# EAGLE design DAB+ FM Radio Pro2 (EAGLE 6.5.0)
AUTHOR: JP Liew; PRODUCT_NAME: DAB+ FM Development Board Pro2; VERSION: 1.5
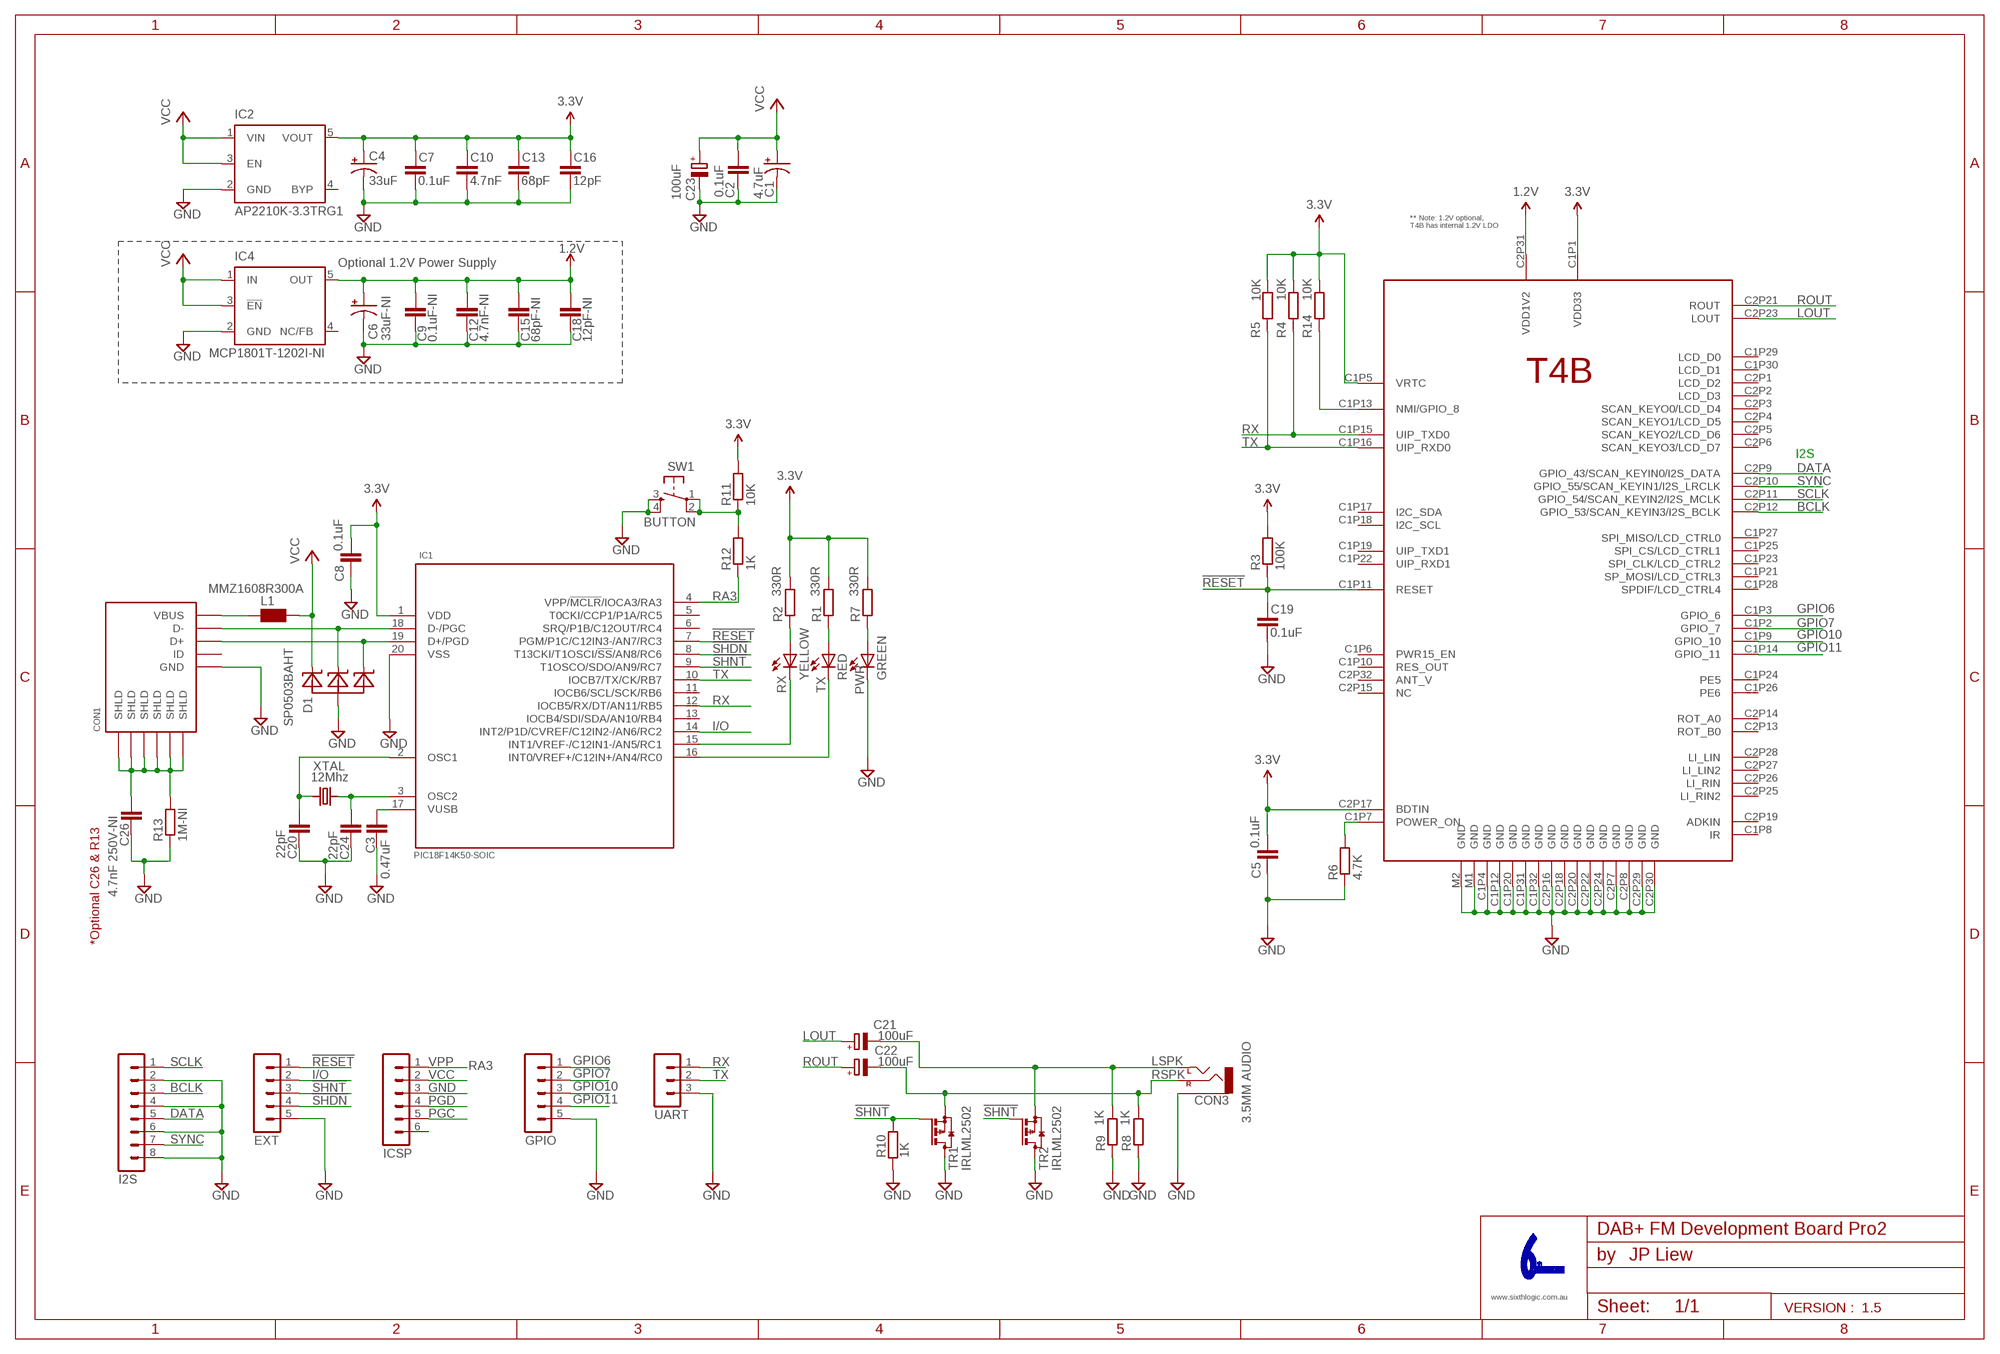
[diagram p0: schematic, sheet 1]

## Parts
C1  4.7uF  CAP_POL1206  [EIA3216]
C2  0.1uF  C-EUC0603  [C0603]
C3  0.47uF  C-EUC0603  [C0603]
C4  33uF  CAP_POL1206  [EIA3216]
C5  0.1uF  C-EUC0603  [C0603]
C6  33uF-NI  CAP_POL1206  [EIA3216]
C7  0.1uF  C-EUC0603  [C0603]
C8  0.1uF  C-EUC0603  [C0603]
C9  0.1uF-NI  C-EUC0603  [C0603]
C10  4.7nF  C-EUC0603  [C0603]
C12  4.7nF-NI  C-EUC0603  [C0603]
C13  68pF  C-EUC0603  [C0603]
C15  68pF-NI  C-EUC0603  [C0603]
C16  12pF  C-EUC0603  [C0603]
C18  12pF-NI  C-EUC0603  [C0603]
C19  0.1uF  C-EUC0603  [C0603]
C20  22pF  C-EUC0603  [C0603]
C21  100uF  CPOL-EUD  [PANASONIC_D]
C22  100uF  CPOL-EUD  [PANASONIC_D]
C23  100uF  CPOL-EUD  [PANASONIC_D]
C24  22pF  C-EUC0603  [C0603]
C26  4.7nF 250V-NI  C-EUC0603  [C0603]
CON1  MicroUSB  CONN_USB-4UCON-11071  [4UCON-11071]
CON3  3.5MM AUDIO  SJ-3523-SMT  [SJ-3523-SMT]
D1  SP0503BAHT  [SOT143]
EXT  MA05-1  [MA05-1]
GPIO  MA05-1  [MA05-1]
I2S  MA08-1  [MA08-1]
IC1  PIC18F14K50-SOIC  [SO20W]
IC2  AP2210K-3.3TRG1  [SOT23-5]
IC4  MCP1801T-1202I-NI  TPS77001  [SOT23-DBV]
ICSP  MA06-1  [MA06-1]
L1  MMZ1608R300A  WE-CBF_0603  [0603]
PWR  GREEN  LEDCHIP-LED0603  [CHIP-LED0603]
R1  330R  R-EU_R0603  [R0603]
R2  330R  R-EU_R0603  [R0603]
R3  100K  R-EU_R0603  [R0603]
R4  10K  R-EU_R0603  [R0603]
R5  10K  R-EU_R0603  [R0603]
R6  4.7K  R-EU_R0603  [R0603]
R7  330R  R-EU_R0603  [R0603]
R8  1K  R-EU_R0603  [R0603]
R9  1K  R-EU_R0603  [R0603]
R10  1K  R-EU_R0603  [R0603]
R11  10K  R-EU_R0603  [R0603]
R12  1K  R-EU_R0603  [R0603]
R13  1M-NI  R-EU_R0603  [R0603]
R14  10K  R-EU_R0603  [R0603]
RX  YELLOW  LEDCHIP-LED0603  [CHIP-LED0603]
SW1  BUTTON  SCHURTER_PUSH_BUTTON  [PUSH_BUTTON_SMD]
TR1  IRLML2502  DMP2305U  [SOT23]
TR2  IRLML2502  DMP2305U  [SOT23]
TX  RED  LEDCHIP-LED0603  [CHIP-LED0603]
U$1  T4B  T4B-SMD  [T4B-SMD]
UART  MA03-1  [MA03-1]
XTAL  12Mhz  CRYSTAL-HC49US  [HC49US-SMD]

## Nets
1.2V: C6.A(+) C9.1 C12.1 C15.1 C18.1 IC4.5(OUT) U$1.C2P31(VDD1V2)
3.3V: C4.A(+) C5.1 C7.1 C8.1 C10.1 C13.1 C16.1 IC1.1(VDD) IC2.5(VOUT) R1.2 R2.2 R3.2 R4.2 R5.2 R7.2 R11.2 R14.2 U$1.C1P1(VDD33) U$1.C1P5(VRTC) U$1.C2P17(BDTIN)
!RESET!: C19.1 EXT.1 IC1.7(PGM/P1C/C12IN3-/AN7/RC3) R3.1 U$1.C1P11(RESET)
!SHDN!: EXT.4 IC1.8(T13CKI/T1OSCI/!SS!/AN8/RC6)
!SHNT!: EXT.3 IC1.9(T1OSCO/SDO/AN9/RC7) R10.2 TR1.1(G) TR2.1(G)
BCLK: I2S.3 U$1.C2P12(GPIO_53/SCAN_KEYIN3/I2S_BCLK)
DATA: I2S.5 U$1.C2P9(GPIO_43/SCAN_KEYIN0/I2S_DATA)
GND: C1.C(-) C2.2 C3.2 C4.C(-) C5.2 C6.C(-) C7.2 C8.2 C9.2 C10.2 C12.2 C13.2 C15.2 C16.2 C18.2 C19.2 C20.2 C23.- C24.2 C26.2 CON1.GND CON3.1(SLEEVE) D1.1 EXT.5 GPIO.5 I2S.2 I2S.4 I2S.6 I2S.8 IC1.20(VSS) IC2.2(GND) IC4.2(GND) ICSP.3 PWR.C R6.1 R8.1 R9.1 R10.1 R13.1 SW1.3 SW1.4 TR1.3(D) TR2.3(D) U$1.C1P4(GND) U$1.C1P12(GND) U$1.C1P20(GND) U$1.C1P31(GND) U$1.C1P32(GND) U$1.C2P7(GND) U$1.C2P8(GND) U$1.C2P16(GND) U$1.C2P18(GND) U$1.C2P20(GND) U$1.C2P22(GND) U$1.C2P24(GND) U$1.C2P29(GND) U$1.C2P30(GND) U$1.M1(GND) U$1.M2(GND) UART.3
GPIO6: GPIO.1 U$1.C1P3(GPIO_6)
GPIO7: GPIO.2 U$1.C1P2(GPIO_7)
GPIO10: GPIO.3 U$1.C1P9(GPIO_10)
GPIO11: GPIO.4 U$1.C1P14(GPIO_11)
I/O: EXT.2 IC1.14(INT2/P1D/CVREF/C12IN2-/AN6/RC2)
LOUT: C21.+ U$1.C2P23(LOUT)
LSPK: C21.- CON3.2(LEFT) R9.2 TR2.2(S)
N$1: PWR.A R7.1
N$2: CON1.VBUS L1.1
N$3: R6.2 U$1.C1P7(POWER_ON)
N$4: IC1.16(INT0/VREF+/C12IN+/AN4/RC0) TX.C
N$5: IC1.15(INT1/VREF-/C12IN1-/AN5/RC1) RX.C
N$6: R14.1 U$1.C1P13(NMI/GPIO_8)
N$7: C3.1 IC1.17(VUSB)
N$8: C26.1 CON1.SHLD@1(SHLD) CON1.SHLD@2(SHLD) CON1.SHLD@3(SHLD) CON1.SHLD@4(SHLD) CON1.SHLD@5(SHLD) CON1.SHLD@6(SHLD) R13.2
N$9: R1.1 TX.A
N$10: R2.1 RX.A
N$11: C20.1 IC1.2(OSC1) XTAL.2
N$12: C24.1 IC1.3(OSC2) XTAL.1
N$13: R11.1 R12.2 SW1.1 SW1.2
PGC: CON1.D- D1.3 IC1.18(D-/PGC) ICSP.5
PGD: CON1.D+ D1.4 IC1.19(D+/PGD) ICSP.4
RA3: IC1.4(VPP/!MCLR!/IOCA3/RA3) ICSP.1 R12.1
ROUT: C22.+ U$1.C2P21(ROUT)
RSPK: C22.- CON3.3(RIGHT) R8.2 TR1.2(S)
RX: IC1.12(IOCB5/RX/DT/AN11/RB5) R4.1 U$1.C1P15(UIP_TXD0) UART.1
SCLK: I2S.1 U$1.C2P11(GPIO_54/SCAN_KEYIN2/I2S_MCLK)
SYNC: I2S.7 U$1.C2P10(GPIO_55/SCAN_KEYIN1/I2S_LRCLK)
TX: IC1.10(IOCB7/TX/CK/RB7) R5.1 U$1.C1P16(UIP_RXD0) UART.2
VCC: C1.A(+) C2.1 C23.+ D1.2 IC2.1(VIN) IC2.3(EN) IC4.1(IN) IC4.3(!EN) ICSP.2 L1.2
Unconnected: CON1.ID IC1.5(T0CKI/CCP1/P1A/RC5) IC1.6(SRQ/P1B/C12OUT/RC4) IC1.11(IOCB6/SCL/SCK/RB6) IC1.13(IOCB4/SDI/SDA/AN10/RB4) IC2.4(BYP) IC4.4(NC/FB) ICSP.6 U$1.C1P6(PWR15_EN) U$1.C1P8(IR) U$1.C1P10(RES_OUT) U$1.C1P17(I2C_SDA) U$1.C1P18(I2C_SCL) U$1.C1P19(UIP_TXD1) U$1.C1P21(SP_MOSI/LCD_CTRL3) U$1.C1P22(UIP_RXD1) U$1.C1P23(SPI_CLK/LCD_CTRL2) U$1.C1P24(PE5) U$1.C1P25(SPI_CS/LCD_CTRL1) U$1.C1P26(PE6) U$1.C1P27(SPI_MISO/LCD_CTRL0) U$1.C1P28(SPDIF/LCD_CTRL4) U$1.C1P29(LCD_D0) U$1.C1P30(LCD_D1) U$1.C2P1(LCD_D2) U$1.C2P2(LCD_D3) U$1.C2P3(SCAN_KEYO0/LCD_D4) U$1.C2P4(SCAN_KEYO1/LCD_D5) U$1.C2P5(SCAN_KEYO2/LCD_D6) U$1.C2P6(SCAN_KEYO3/LCD_D7) U$1.C2P13(ROT_B0) U$1.C2P14(ROT_A0) U$1.C2P15(NC) U$1.C2P19(ADKIN) U$1.C2P25(LI_RIN2) U$1.C2P26(LI_RIN) U$1.C2P27(LI_LIN2) U$1.C2P28(LI_LIN) U$1.C2P32(ANT_V)

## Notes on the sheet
- ** Note: 1.2V optional, 
  T4B has internal 1.2V LDO
- Optional 1.2V Power Supply
- I2S
- *Optional C26 & R13
- VPP
- www.sixthlogic.com.au

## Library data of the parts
C1 C4 C6 = SparkFun:CAP_POL: Capacitor Polarized
C2 C3 C5 C7-C10 C12 C13 C15 C16 C18-C20 C24 C26 = rcl:C-EU: CAPACITOR, European symbol
C21-C23 = rcl:CPOL-EU: POLARIZED CAPACITOR, European symbol
CON1 = SixthLogic:CONN_USB: USB Connector; DESCRIPTION: B TYPE FEMALE 05P SMT 90° WITHOUT POST 2 SHELL TABS; MF: 4UCON; MPN: 11071; URL: http://www.4uconnector.com/online/Itemadrawing.asp?fldseries=11071&seriesno_a=1006
CON3 = Monkey:SJ-3523-SMT: SERIES: SJ-352X-SMT ? DESCRIPTION: 3.5 MM AUDIO JACKS http://products.cui.com/getpdf.aspx?fileID=7777
D1 = Monkey:SP0503BAHT: Surface Mount TVS Avalanche Diode Array http://www.littelfuse.com/data/en/Data_Sheets/SP05x_LeadFree.pdf
EXT GPIO = con-lstb:MA05-1: PIN HEADER; OC_FARNELL: unknown; OC_NEWARK: unknown
I2S = con-lstb:MA08-1: PIN HEADER; OC_FARNELL: unknown; OC_NEWARK: unknown
IC1 = Monkey:PIC18F14K50: PIC18F/LF1XK50 20-Pin USB Flash Microcontrollers with nanoWatt XLP Technology. PIC18F13K50, PIC18LF13K50, PIC18F14K50, PIC18LF14K50. From: http://ww1.microchip.com/downloads/en/DeviceDoc/41350E.pdf
IC2 = SixthLogic:AP2210K: The AP2210 is a 300mA ULDO regulator which provides very low noise, ultra low dropout voltage (typically 250mV at 300mA), very low standby current (1μA maximum) and excellent power supply ripple rejection (PSRR 75dB at 100Hz) in battery powered applications, such as handsets, PDAs and in noise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; DESCRIPTION: IC REG LDO 3.3V 0.3A SOT23-5; MF: Diodes Inc; MPN: AP2210K-3.3TRG1; OC_DIGIKEY: AP2210K-3.3TRG1DITR-ND; URL: https://www.digikey.com/product-detail/en/diodes-incorporated/AP2210K-3.3TRG1/AP2210K-3.3TRG1DITR-ND/4470819
IC4 = texas:TPS770*: ULTRALOW-POWER 50-mA LOW-DROPOUT LINEAR REGULATORS 50-mA Low-Dropout Regulator Source: http://focus.ti.com/lit/ds/symlink/tps77001.pdf; MF: TEXAS INSTRUMENTS; MPN: TPS77001DBVT; OC_FARNELL: 8461554; OC_NEWARK: 77C1171
ICSP = con-lstb:MA06-1: PIN HEADER; OC_FARNELL: unknown; OC_NEWARK: unknown
L1 = wuerth-elektronik:WE-CBF: SMD EMI Suppression Ferrite Beads
PWR RX TX = led:LED: LED
R1-R10 R14 = rcl:R-EU_: RESISTOR, European symbol
R11-R13 = resistor:R-EU_: RESISTOR, European symbol
SW1 = Monkey:SCHURTER_PUSH_BUTTON: SCHURTER - 1301.9316 - SWITCH, SMD, PUSH, 7MM Datasheet : http://www.schurterinc.com/pdf/english/typ_lph.pdf
TR1 TR2 = transistor-small-signal:DMP2305U
U$1 = SixthLogic:T4B
UART = con-lstb:MA03-1: PIN HEADER; OC_FARNELL: unknown; OC_NEWARK: unknown
XTAL = SixthLogic:CRYSTAL: 2 pin Crystal

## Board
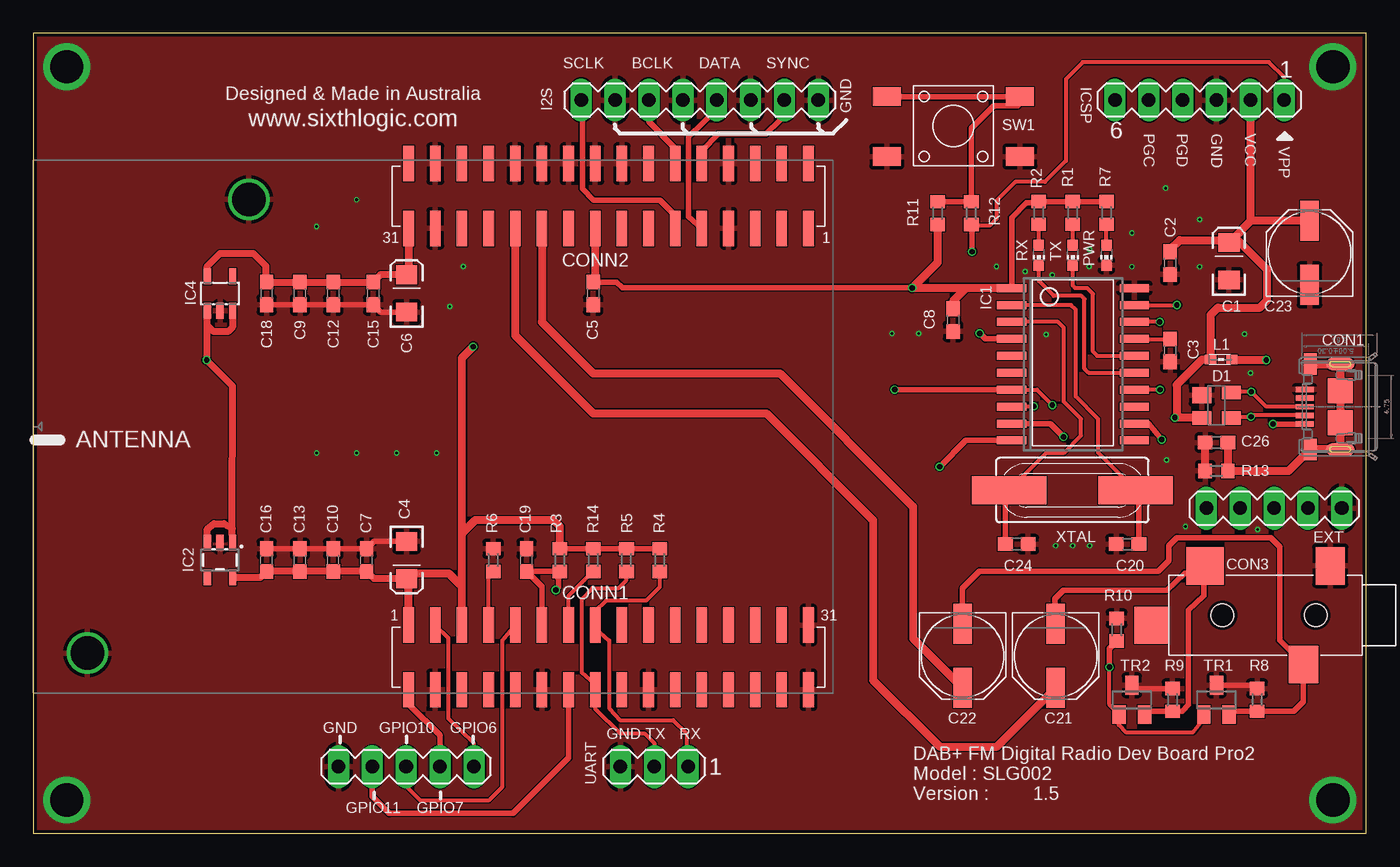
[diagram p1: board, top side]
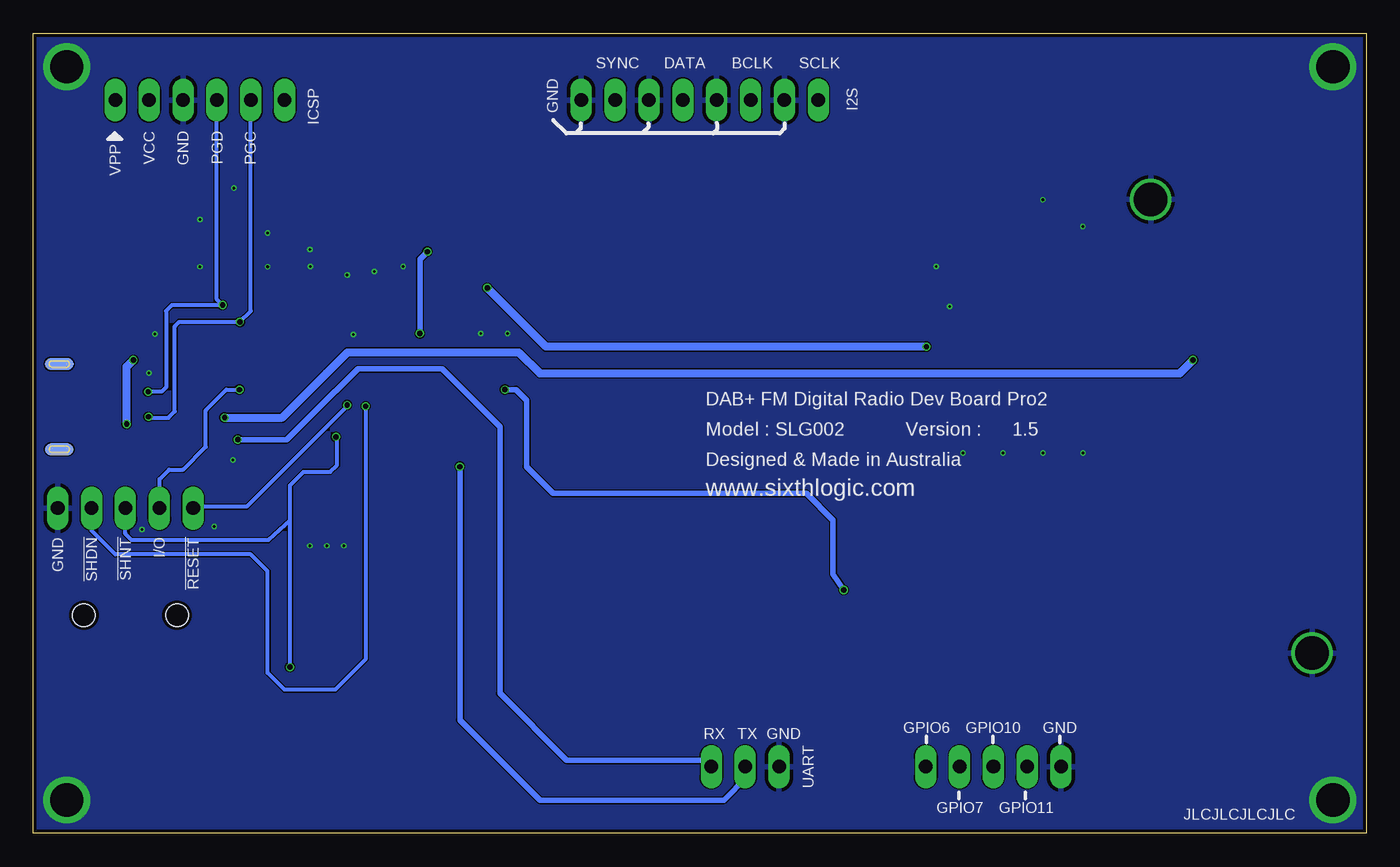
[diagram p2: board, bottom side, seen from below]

Size 100 x 60 mm. Coordinates in mm from the lower left corner, seen from the top.
Outline: 0,0 100,0 100,60 0,60 0,0
Copper layers (1*16): Top 0.035mm / dielectric 1.5mm / Bottom 0.035mm
Design rules "GeekAmmo *": minimum track width 12mil, minimum drill 0.2mm, track to track 3.5mil, track to pad 3.5mil, pad to pad 3.5mil, via to via 3.5mil, smd to smd 3.5mil, copper to edge 10mil, drill to drill 8mil, minimum pad ring 12mil, minimum via ring 4mil, stop-mask expansion 4mil, vias tented up to drill 25mil, thermal gap 10mil
tRestrict: area 13.5,22 to 14.5,22.5; area 95,33 to 95.7,33.2

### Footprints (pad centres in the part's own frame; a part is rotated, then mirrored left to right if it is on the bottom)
EIA3216 = smd 1.4 x 1.6: A 1.4,0; C -1.4,0
C0603 = smd 1.1 x 1: 1 -0.85,0; 2 0.85,0
PANASONIC_D = smd 3 x 1.4: + 2.4,0; - -2.4,0
4UCON-11071 = smd 0.4 x 1.35: D+ 0,4.125; D- -0.65,4.125; GND 1.3,4.125; ID 0.65,4.125; VBUS -1.3,4.125 | smd 1.9 x 1.9: SHLD@1 -1.2,1.45; SHLD@2 1.2,1.45 | smd 1.6 x 1: SHLD@3 -3.2,3.7; SHLD@4 3.2,3.7 | smd 0.9 x 2.15: SHLD@5 -3.2,1.45; SHLD@6 3.2,1.45 | smd 0.9 x 2.15 bottom: SHLD@7 -3.2,1.45; SHLD@8 3.2,1.45
SJ-3523-SMT = smd 2.2 x 2.8: 1 -1.1,-3.7; 3 0.9,3.7 | smd 2.8 x 2.8: 2 8.3,-3.7 | smd 2.6 x 2.8: 10 12.3,0.75 | hole 1.7: 0,0; 7,0
SOT143 = smd 1.2 x 1.44: 1 -0.75,-1.1 | smd 1 x 1.44: 2 0.95,-1.1; 3 0.95,1.1; 4 -0.95,1.1
MA05-1 = drill 1.016 long: 1 -5.08,0; 2 -2.54,0; 3 0,0; 4 2.54,0; 5 5.08,0
MA08-1 = drill 1.016 long: 1 -8.89,0; 2 -6.35,0; 3 -3.81,0; 4 -1.27,0; 5 1.27,0; 6 3.81,0; 7 6.35,0; 8 8.89,0
SO20W = smd 0.6 x 2.2: 1 -5.715,-4.6; 2 -4.445,-4.6; 3 -3.175,-4.6; 4 -1.905,-4.6; 5 -0.635,-4.6; 6 0.635,-4.6; 7 1.905,-4.6; 8 3.175,-4.6; 9 4.445,-4.6; 10 5.715,-4.6; 11 5.715,4.6; 12 4.445,4.6; 13 3.175,4.6; 14 1.905,4.6; 15 0.635,4.6; 16 -0.635,4.6; 17 -1.905,4.6; 18 -3.175,4.6; 19 -4.445,4.6; 20 -5.715,4.6
SOT23-5 = smd 0.55 x 1.2: 1 -0.95,-1.3; 2 0,-1.3; 3 0.95,-1.3; 4 0.95,1.3; 5 -0.95,1.3
SOT23-DBV = smd 0.55 x 1.2: 1 -0.95,-1.3; 2 0,-1.3; 3 0.95,-1.3; 4 0.95,1.3; 5 -0.95,1.3
MA06-1 = drill 1.016 long: 1 -6.35,0; 2 -3.81,0; 3 -1.27,0; 4 1.27,0; 5 3.81,0; 6 6.35,0
0603 = smd 0.85 x 0.7: 1 -0.9,0; 2 0.7,0
CHIP-LED0603 = smd 0.8 x 0.8: A 0,-0.75; C 0,0.75
R0603 = smd 1 x 1.1: 1 -0.85,0; 2 0.85,0
PUSH_BUTTON_SMD = smd 2.1 x 1.4: 1 0,4.5; 2 10,4.5; 3 0,0; 4 10,0
SOT23 = smd 1 x 1.4: 1 -0.95,-1.1; 2 0.95,-1.1; 3 0,1.1
T4B-SMD = smd 0.8 x 2.65: C1P1 28.16,5.125; C1P2 28.16,0.275; C1P3 30.16,5.125; C1P4 30.16,0.275; C1P5 32.16,5.125; C1P6 32.16,0.275; C1P7 34.16,5.125; C1P8 34.16,0.275; C1P9 36.16,5.125; C1P10 36.16,0.275; C1P11 38.16,5.125; C1P12 38.16,0.275; C1P13 40.16,5.125; C1P14 40.16,0.275; C1P15 42.16,5.125; C1P16 42.16,0.275; C1P17 44.16,5.125; C1P18 44.16,0.275; C1P19 46.16,5.125; C1P20 46.16,0.275; C1P21 48.16,5.125; C1P22 48.16,0.275; C1P23 50.16,5.125; C1P24 50.16,0.275; C1P25 52.16,5.125; C1P26 52.16,0.275; C1P27 54.16,5.125; C1P28 54.16,0.275; C1P29 56.16,5.125; C1P30 56.16,0.275; C1P31 58.16,5.125; C1P32 58.16,0.275; C2P1 58.16,34.875; C2P2 58.16,39.725; C2P3 56.16,34.875; C2P4 56.16,39.725; C2P5 54.16,34.875; C2P6 54.16,39.725; C2P7 52.16,34.875; C2P8 52.16,39.725; C2P9 50.16,34.875; C2P10 50.16,39.725; C2P11 48.16,34.875; C2P12 48.16,39.725; C2P13 46.16,34.875; C2P14 46.16,39.725; C2P15 44.16,34.875; C2P16 44.16,39.725; C2P17 42.16,34.875; C2P18 42.16,39.725; C2P19 40.16,34.875; C2P20 40.16,39.725; C2P21 38.16,34.875; C2P22 38.16,39.725; C2P23 36.16,34.875; C2P24 36.16,39.725; C2P25 34.16,34.875; C2P26 34.16,39.725; C2P27 32.16,34.875; C2P28 32.16,39.725; C2P29 30.16,34.875; C2P30 30.16,39.725; C2P31 28.16,34.875; C2P32 28.16,39.725 | drill 2.5: M1 4.06,3.02; M2 16.17,37.04
MA03-1 = drill 1.016 long: 1 -2.54,0; 2 0,0; 3 2.54,0
HC49US-SMD = smd 5.6 x 2.1: 1 -4.75,0; 2 4.75,0

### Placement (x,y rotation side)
C1  89.71,42.9 90 top
C2  85.29,42.77 270 top
C3  85.29,36.22 270 top
C4  28,20.5 270 top
C5  42,40.5 270 top
C6  28,40.5 90 top
C7  25,20.5 90 top
C8  69,38.5 270 top
C9  20,40.5 270 top
C10  22.5,20.5 90 top
C12  22.5,40.5 270 top
C13  20,20.5 90 top
C15  25.5,40.5 270 top
C16  17.5,20.5 90 top
C18  17.5,40.5 270 top
C19  37,20.5 90 top
C20  82.09,21.69 180 top
C21  76.7,13.31 270 top
C22  69.72,13.31 270 top
C23  95.75,43.54 90 top
C24  73.78,21.69 0 top
C26  88.77,29.31 180 top
CON1  99.5,32 90 top
CON3  96.21,16.36 180 top
D1  88.77,32.11 270 top
EXT  93.09,24.38 0 top
GPIO  27.97,5 180 top
I2S  50,55 0 top
IC1  78,35.18 270 top
IC2  14,20.5 180 top
IC4  14,40.49 0 top
ICSP  87.5,55 180 top
L1  89.02,35.53 180 top
PWR  80.52,43.36 180 top
R1  77.97,46.53 90 top
R2  75.44,46.53 90 top
R3  39.5,20.5 90 top
R4  47,20.5 90 top
R5  44.5,20.5 90 top
R6  34.5,20.5 270 top
R7  80.52,46.53 90 top
R8  91.82,10.01 270 top
R9  85.47,10.01 270 top
R10  81.28,15.27 270 top
R11  67.84,46.52 270 top
R12  70.38,46.52 90 top
R13  88.77,27.18 0 top
R14  42,20.5 90 top
RX  75.44,43.36 180 top
SW1  64.03,50.76 0 top
TR1  88.77,10.01 0 top
TR2  82.42,10.01 0 top
TX  77.97,43.36 180 top
U$1  0,10.5 0 top
UART  46.59,5 180 top
XTAL  77.96,25.74 0 top

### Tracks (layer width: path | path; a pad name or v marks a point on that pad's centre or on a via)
1.2V
  Top 0.406: 17.45,41.4 C18.1
  Top 0.508: C18.1 C9.1 C12.1 C15.1 26.05,41.9 C6.A | IC4.5 13.05,42.55 14,43.5 16.51,43.5 17.45,42.56 17.45,41.4
  Top 0.61: U$1.C2P31 28.16,42.06 C6.A
3.3V  (via drill 0.4)
  Top 0.406: R2.2 R1.2 R7.2 | R2.2 75.4,47.35 | IC1.1 73.4,46.18 74.52,47.31 75.36,47.31 R2.2 | R3.2 R14.2 R5.2 R4.2 | v65.94,40.91 44.2,40.91 43.76,41.34 42.01,41.34 C5.1
  Top 0.508: C4.A 25.55,19.1 C7.1 C10.1 C13.1 C16.1 17.05,19.2 IC2.5
  Top 0.61: 70,40.91 v65.94,40.91 67.84,42.81 R11.2 | 70,40.91 73.39,40.91 IC1.1 | C8.1 69,39.91 70,40.91 | C4.A 28.16,18.94 U$1.C1P1 28.16,19.34 28,19.5 31.16,19.5 32.16,18.5 | U$1.C1P5 32.16,18.5 | 32.16,18.5 32.16,22.5 | 32.16,22.5 32.16,35.66 v33,36.5 | R3.2 39.5,23 39,23.5 33.16,23.5 32.16,22.5 | U$1.C2P17 42.16,41.51 C5.1
  Bottom 0.61: v33,36.5 61.53,36.5 v65.94,40.91
!RESET!  (via drill 0.4)
  Top 0.305: IC1.7 75.3,33.27 v76.45,32.12
  Top 0.406: R3.1 C19.1 38.16,18.49 U$1.C1P11 | IC1.7 v64.63,33.27 v64.62,33.28 | 39.4,19.25 39.4,18.45 v39.2,18.25
  Top 0.61: 39.4,19.25 39.4,19.55 R3.1
  Bottom 0.305: v76.45,32.12 76.45,32.05 84,24.5 87.89,24.5 EXT.1
  Bottom 0.406: v64.62,33.28 63.78,33.28 63,32.5 63,27.5 61,25.5 42,25.5 40,23.5 40,19.45 v39.2,18.25
!SHDN!  (via drill 0.4)
  Top 0.305: v75.07,32.03 73.43,32.03 IC1.8
  Bottom 0.305: EXT.4 95.63,22.71 93.85,20.93 83.69,20.93 82.42,19.66 82.42,12.04 81.15,10.77 77.34,10.77 75.07,13.04 v75.07,32.03
!SHNT!  (via drill 0.4)
  Top 0.305: v80.74,12.47 80.74,9.63 TR2.1 81.43,8.87 81.43,8.13 81.96,7.59 87.02,7.59 87.82,8.57 TR1.1
  Top 0.406: TR2.1 81.22,9.16 | v80.74,12.47 80.72,12.5 80.72,13.86 R10.2 | IC1.9 76.29,30.73 v77.29,29.73
  Bottom 0.305: v80.74,12.47 80.74,23.47 | 80.74,23.47 80.74,26.09 79.73,27.11 77.73,27.11 77.22,27.62 77.22,29.66 v77.29,29.73 | 80.74,23.47 82.37,22 92.61,22 93.09,22.48 EXT.3
BCLK
  Top 0.406: U$1.C2P12 48.16,51.37 46.18,53.35 46.18,54.99 I2S.3
DATA
  Top 0.305: U$1.C2P9 50.12,45.38 | 51.3,54.97 I2S.5
  Top 0.406: 50.12,45.38 49.17,46.25 49.17,52.25 51.3,54.3 51.3,54.97
GND  (via drill 0.2, 2.5)
  Top 0.406: TR1.3 91.57,11.11 R8.1 | R9.1 82.67,10.86 TR2.3 | C18.2 C9.2 C12.2 C15.2 26.05,39.1 C6.C | C16.2 C13.2 C10.2 C7.2 25.55,21.9 C4.C
  Top 0.61: R13.1 C26.2
  other vias: 97.5,57.5 97.5,2.5 77.97,21.57 76.7,21.57 79.25,21.57 82.42,45.03 79.25,43.79 79.22,42.52 74.42,42.14 87.5,46.03 87.5,42.49 91.34,34.52 85.03,28 90.88,37.44 76.45,41.88 82.42,42.49 84.96,48.39 72.26,42.52 86.43,23.01 91.84,22.78 2.5,57.5 64.42,37.49 66.42,37.49 75.98,37.42 21.26,28.52 24.26,28.52 27.26,28.52 30.26,28.52 32.26,42.52 31.26,39.52 21.26,45.52 24.26,47.52 2.5,2.5
  pour Top: -23,67 -23,-19 123,-19 123,67
  pour Bottom: -25,68 -25,-20 125,-20 125,68
GPIO6
  Top 0.305: GPIO.1 33.05,6.75 31.15,8.6 31.15,14.63 U$1.C1P3
GPIO7
  Top 0.406: U$1.C1P2 28.16,9.69 30.5,7.35 GPIO.2
GPIO10
  Top 0.305: GPIO.3 27.97,3.53 29,2.5 34.2,2.5 35.2,3.5 35.2,14.46 U$1.C1P9
GPIO11
  Top 0.406: U$1.C1P14 40.16,5.66 36,1.5 26.7,1.5 25.4,2.8 25.4,4.97 GPIO.4
I/O  (via drill 0.4)
  Top 0.305: v84.53,33.27 IC1.14
  Bottom 0.305: EXT.2 90.52,24.41 90.52,26.57 89.81,27.28 88.77,27.28 87.07,28.98 87.07,31.73 85.52,33.27 v84.53,33.27
LOUT
  Top 0.61: C21.+ 72.3,6.5 68,6.5 63,11.5 63,23.5 55,31.5 42,31.5 36.16,37.34 U$1.C2P23
LSPK
  Top 0.305: CON3.2 87.83,19.82
  Top 0.406: TR2.2 83.62,9.16 R9.2 86.19,9.16 86.66,9.63 86.66,16.71 87.83,17.83 87.83,19.82 | CON3.2 87.54,19.53 86.38,19.51 85.06,18.24 77.29,18.24 76.63,17.58 76.63,15.79 C21.-
N$1
  Top 0.305: PWR.A R7.1
N$2  (via drill 0.4)
  Top 0.305: 89.96,35.5 L1.1
  Top 0.406: CON1.VBUS v93,30.7
  Top 0.61: v92.5,35.5 89.96,35.5
  Bottom 0.61: v93,30.7 93,35 v92.5,35.5
N$3
  Top 0.305: U$1.C1P7 34.16,19.31 R6.2
N$4
  Top 0.305: TX.C 77.97,41.1 78.18,40.89 79.07,40.89 79.5,40.46 79.5,36.15 79.83,35.81 IC1.16
N$5
  Top 0.305: RX.C 75.44,41.43 76.55,40.31 78.64,40.31 78.86,40.08 78.86,34.85 79.17,34.54 IC1.15
N$6
  Top 0.305: U$1.C1P13 40.16,17.81 R14.1
N$7
  Top 0.305: C3.1 82.61,37.07 IC1.17
N$8
  Top 0.61: C26.1 R13.2 94.18,27.18 CON1.SHLD@3 CON1.SHLD@5 CON1.SHLD@1 CON1.SHLD@2 CON1.SHLD@6 CON1.SHLD@4
N$9
  Top 0.305: 77.97,45.9 R1.1 TX.A
N$10
  Top 0.305: 75.44,45.9 R2.1 RX.A
N$11
  Top 0.305: IC1.2 77.85,39.62 78.2,39.27 78.2,32.77 79.88,31.09 79.88,28.57 XTAL.2
  Top 0.406: C20.1 82.94,25.51 XTAL.2
N$12
  Top 0.305: IC1.3 76.88,38.35 77.31,37.92 77.31,32.38 78.61,31.09 78.61,29.82 77.34,28.55 76.07,28.55 | 76.07,28.55 76.07,28.54 | 76.07,28.55 76.02,28.55 XTAL.1
  Top 0.406: C24.1 72.93,25.46 XTAL.1
N$13
  Top 0.406: R11.1 R12.2 70.38,52.87 72.08,54.57 73.87,54.57 SW1.2 SW1.1
PGC  (via drill 0.4)
  Top 0.305: v84.5,38.35 IC1.18 | D1.3 89.96,31.24 v91.36,31.24 91.47,31.35 CON1.D-
  Bottom 0.305: v91.36,31.24 91.27,31.16 D1.3 89.38,31.65 89.38,38.02 89.05,38.35 v84.5,38.35 83.69,39.17 ICSP.5
PGD  (via drill 0.4)
  Top 0.305: IC1.19 v85.8,39.62 | D1.4 89.94,33.12 v91.39,33.12 92.51,32 CON1.D+
  Bottom 0.305: v91.39,33.12 90.37,33.12 90.04,33.45 90.04,39.19 89.61,39.62 v85.8,39.62 86.23,40.06 ICSP.4
RA3  (via drill 0.4)
  Top 0.305: ICSP.1 93.85,56.7 92.71,57.84 78.74,57.84 77.47,56.57 77.47,50.43 75.89,48.85 73.69,48.85 72.26,47.43 72.26,46.09 71.75,45.58 70.47,45.58 R12.1
  Top 0.406: IC1.4 71.42,37.08 v71,37.5 | v70.43,43.62 70.43,45.62 R12.1
  Bottom 0.406: v71,37.5 71,43.06 v70.43,43.62
ROUT
  Top 0.61: C22.+ 66,14.63 66,24.5 56,34.5 42,34.5 38.16,38.34 U$1.C2P21
RSPK
  Top 0.406: CON3.3 95.3,12.49 95.3,9.88 94.58,9.16 R8.2 89.72,9.16 TR1.2 | 95.35,12.54 CON3.3 | C22.- 69.72,18.39 70.99,19.66 84.4,19.66 85.19,20.45 85.19,21.57 85.8,22.18 92.83,22.18 93.5,21.5 93.5,14.47 CON3.3
RX  (via drill 0.4)
  Top 0.305: UART.1 49,5.13 49,7.5 48,8.5 44,8.5 43.2,9.4 43.2,14.45 42.16,15.39 U$1.C1P15 42.16,16.66 43,17.5 46,17.5 47,18.5 R4.1
  Top 0.406: IC1.12 83.68,30.73 v84.66,29.53
  Bottom 0.406: v84.66,29.53 80.97,29.53 77.34,33.16 77.32,33.16 75.64,34.83 69.33,34.83 65,30.5 65,10.5 60,5.5 49.63,5.5 UART.1
SCLK
  Top 0.406: U$1.C2P11 48.16,46.34 47,47.5 42.05,47.5 41.2,48.35 41.2,54.91 I2S.1
SYNC
  Top 0.406: U$1.C2P10 50.16,51.21 51.4,52.45 54.95,52.45 56,53.5 56,54.65 I2S.7
TX  (via drill 0.4)
  Top 0.305: UART.2 46.6,6.75 45.85,7.5 44,7.5 42.16,9.34 U$1.C1P16 42.16,11.19 41.15,12.05 41.15,17.55 41.95,18.4 43.9,18.4 44.5,19 R5.1
  Top 0.406: IC1.10 69.96,29.46 v68,27.5
  Bottom 0.406: v68,27.5 68,8.5 62,2.5 48.2,2.5 46.5,4.2 46.5,4.91 UART.2
VCC  (via drill 0.4)
  Top 0.305: D1.2 87.73,31.1
  Top 0.406: L1.2 88.34,35.51 | 89.73,44.32 C1.A | C1.A 89.41,44.6 | C1.A 89.66,44.35 | 13,39.14 IC4.1 | C2.1 85.29,43.79 | 89.51,44.5 C1.A
  Top 0.508: IC2.1 14.93,22.87 | 14.93,22.87 14.95,33.55 v13,35.5 13.05,35.5 13.05,38.11 | 13.05,38.11 IC4.1 | IC4.3 14.95,37.97 14.61,37.63 13.53,37.63 13.05,38.11 | IC2.3 13.05,22.84 13.54,23.23 14.31,23.23 14.93,22.87
  Top 0.61: 88.34,35.51 88.34,38.89 88.87,39.42 92.02,39.42 92.58,39.98 92.58,42.27 90.13,44.72 | D1.2 85.67,31.16 v85.65,31.18 85.78,31.3 85.78,33.64 87.67,35.53 L1.2 | 85.29,43.79 86,44.5 89.51,44.5 | ICSP.2 91.31,45.9 | 91.31,45.9 90.13,44.72 | 90.13,44.72 C1.A | C23.+ 91.34,45.94 91.31,45.9
  Bottom 0.61: v85.65,31.18 81.32,31.18 78,34.5 78,34.51 76.43,36.08 63.58,36.08 62,34.5 14,34.5 v13,35.5

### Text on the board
tPlace: SCLK | BCLK | DATA | SYNC | Designed & Made in Australia | I2S | GND | www.sixthlogic.com | PGC | PGD | GND | VCC | VPP | GND | GPIO10 | GPIO6 | GND | TX | RX | DAB+ FM Digital Radio Dev Board Pro2 | UART | Model : SLG002 | GPIO11 | GPIO7 | Version :
bPlace: SCLK | BCLK | DATA | SYNC | ICSP | GND | PGC | PGD | GND | VCC | VPP | DAB+ FM Digital Radio Dev Board Pro2 | Version : | Model : SLG002 | Designed & Made in Australia | www.sixthlogic.com | !RESET! | I/O | !SHNT! | !SHDN! | GND | GND | GPIO10 | GPIO6 | GND | TX | RX | GPIO11 | GPIO7 | JLCJLCJLCJLC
